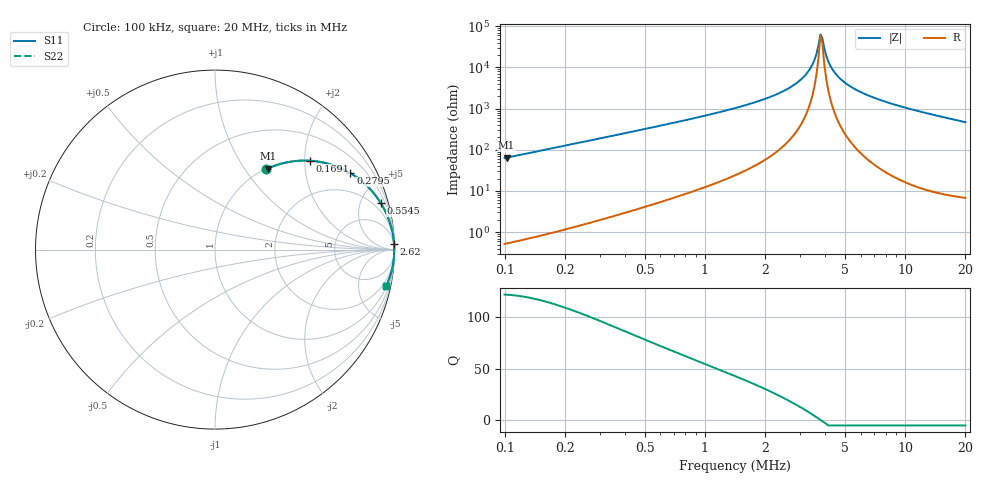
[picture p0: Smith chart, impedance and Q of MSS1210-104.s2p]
# MHz S MA R 50
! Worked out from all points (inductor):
!   233 points, 100 kHz to 20 MHz, reference 50 ohm
!   read as one part in series: L = 100 uH near 102.3 kHz
!   highest Q = 121 at 102.3 kHz (marker M1), where L = 100 uH
!   self-resonance near 3.776 MHz
!   S11 on the Smith chart (normalised r, x): 100 kHz: 1.01, +1.26; 169.1 kHz: 1.02, +2.13; 279.5 kHz: 1.04, +3.53; 554.5 kHz: 1.10, +7.10; 2.62 MHz: 4, +62; 20 MHz: 1.14, -9.38
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0.1  0.5303 57.5  0.8434 -32.0  0.8434 -32.0  0.5303 57.5
0.10231  0.539 56.9  0.8379 -32.6  0.8379 -32.6  0.539 56.9
0.1690906  0.7254 43.0  0.682 -46.5  0.682 -46.5  0.7254 43.0
0.2436751  0.8342 32.9  0.5434 -56.5  0.5434 -56.5  0.8342 32.9
0.2794605  0.866 29.4  0.4913 -60.0  0.4913 -60.0  0.866 29.4
0.5544565  0.9592 15.7  0.2702 -73.6  0.2702 -73.6  0.9592 15.7
0.5937753  0.964 14.6  0.2528 -74.6  0.2528 -74.6  0.964 14.6
1.446882  0.9934 5.4  0.09384 -83.3  0.09384 -83.3  0.9934 5.4
2.038012  0.9966 3.2  0.05575 -84.9  0.05575 -84.9  0.9966 3.2
2.620036  0.9978 1.8  0.03204 -85.2  0.03204 -85.2  0.9978 1.8
3.07422  0.9983 1.0  0.01808 -84.0  0.01808 -84.0  0.9983 1.0
3.446086  0.9985 0.5  0.008443 -79.3  0.008443 -79.3  0.9985 0.5
3.607136  0.9985 0.3  0.004701 -71.5  0.004701 -71.5  0.9985 0.3
3.775713  0.9986 0.0  0.001579 -23.4  0.001579 -23.4  0.9986 0.0
3.862934  0.9986 -0.1  0.00193 41.8  0.00193 41.8  0.9986 -0.1
3.952169  0.9986 -0.2  0.003509 65.8  0.003509 65.8  0.9986 -0.2
4.136871  0.9986 -0.4  0.007188 78.3  0.007188 78.3  0.9986 -0.4
4.430234  0.9985 -0.7  0.01292 83.2  0.01292 83.2  0.9985 -0.7
4.7444  0.9985 -1.1  0.01874 84.8  0.01874 84.8  0.9985 -1.1
5.961611  0.9979 -2.2  0.03901 85.9  0.03901 85.9  0.9979 -2.2
8.397251  0.996 -4.2  0.07349 84.7  0.07349 84.7  0.996 -4.2
20  0.9752 -12.0  0.2078 77.2  0.2078 77.2  0.9752 -12.0
